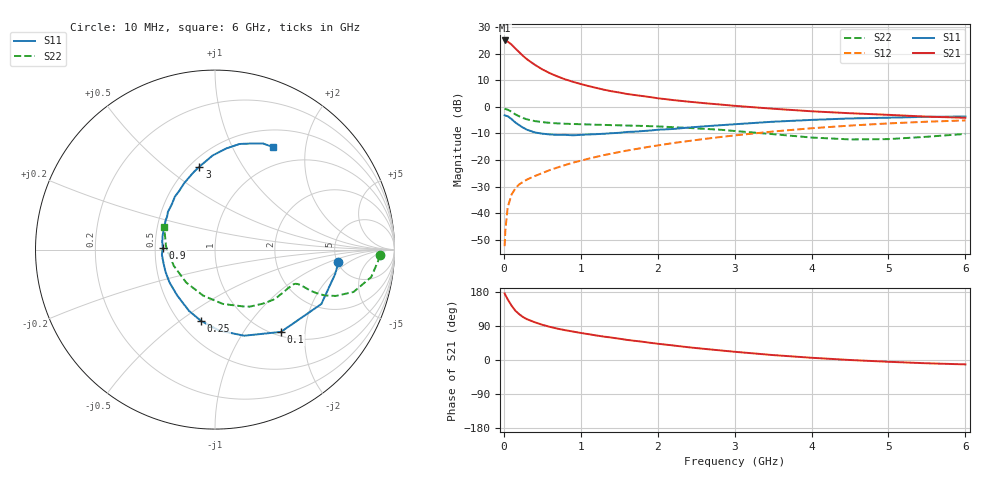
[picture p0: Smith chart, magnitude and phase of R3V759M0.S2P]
! SIEMENS Small Signal Semiconductors
! BFR181
! Si NPN RF Bipolar Junction Transistor in SOT23
! VCE = 0.75 V  IC = 9 mA
! Common Emitter S-Parameters:  May  1996
# GHz  S  MA  R  50
!  f  S11  S21  S12  S22
! GHz  MAG  ANG  MAG  ANG  MAG  ANG  MAG  ANG
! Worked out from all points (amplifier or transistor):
!   36 points, 10 MHz to 6 GHz, reference 50 ohm
!   highest |S21| = 24.9 dB at 10 MHz (marker M1)
!   |S21| within 3 dB of that: start of sweep to 149.3 MHz
!   unconditionally stable (mu >= 1): start of sweep to 10.57 MHz; 362.7 MHz to end of sweep
!   at 250 MHz: K = 0.81, MSG = 23.7 dB, |S12| = -28.2 dB
!   at 1.4 GHz: K = 1.37, MAG = 8.1 dB, |S12| = -17.6 dB
!   at 6 GHz: K = 1.08, MAG = -1.3 dB, |S12| = -5.1 dB
!   S11 on the Smith chart (normalised r, x): 10 MHz: 5.11, -1.37; 100 MHz: 1.07, -1.50; 250 MHz: 0.63, -0.60; 900 MHz: 0.55, +0.01; 3 GHz: 0.56, +0.66; 6 GHz: 0.72, +1.45
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0.01  0.6916 -5.8  17.67 175.9  0.0024 79.1  0.92 -2.0
0.02  0.6831 -11.5  17.55 171.5  0.0048 81.7  0.9101 -4.2
0.05  0.6655 -27.1  16.84 160.1  0.0129 75.6  0.8834 -10.0
0.1  0.5876 -51.3  14.79 143.5  0.0224 68.2  0.8071 -17.0
0.15  0.5065 -71.3  12.48 130.0  0.0293 61.8  0.7205 -21.0
0.2  0.452 -86.9  10.63 120.9  0.0349 59.3  0.662 -22.7
0.25  0.4054 -100.9  9.046 113.3  0.0388 57.9  0.6153 -23.2
0.3  0.371 -113.0  7.847 107.7  0.0429 58.0  0.5809 -23.3
0.4  0.3306 -129.8  6.2 99.8  0.0498 58.8  0.5396 -22.8
0.5  0.3125 -144.3  5.055 92.9  0.0568 60.6  0.5153 -22.5
0.6  0.3022 -156.1  4.271 87.4  0.0649 62.1  0.4988 -22.6
0.7  0.2964 -166.3  3.711 82.6  0.0725 63.3  0.4877 -23.0
0.9  0.291 178.3  2.947 75.0  0.0894 64.4  0.4752 -24.4
1.1  0.302 165.1  2.456 68.2  0.1058 65.4  0.4659 -26.6
1.3  0.3112 154.6  2.099 61.8  0.1235 65.4  0.457 -29.1
1.6  0.3366 141.1  1.744 53.1  0.1504 64.6  0.4446 -33.7
2.2  0.3831 121.3  1.339 38.4  0.2082 61.2  0.4137 -44.8
3  0.4699 100.7  1.044 21.7  0.2897 53.7  0.3512 -64.2
3.5  0.5243 91.5  0.92 13.0  0.3433 48.1  0.3059 -81.8
4.5  0.6042 76.9  0.757 0.0  0.4434 34.7  0.2437 -131.2
5.5  0.6487 65.8  0.653 -8.7  0.5246 20.3  0.2735 176.2
6  0.656 60.7  0.622 -11.6  0.555 13.0  0.3095 156.1
